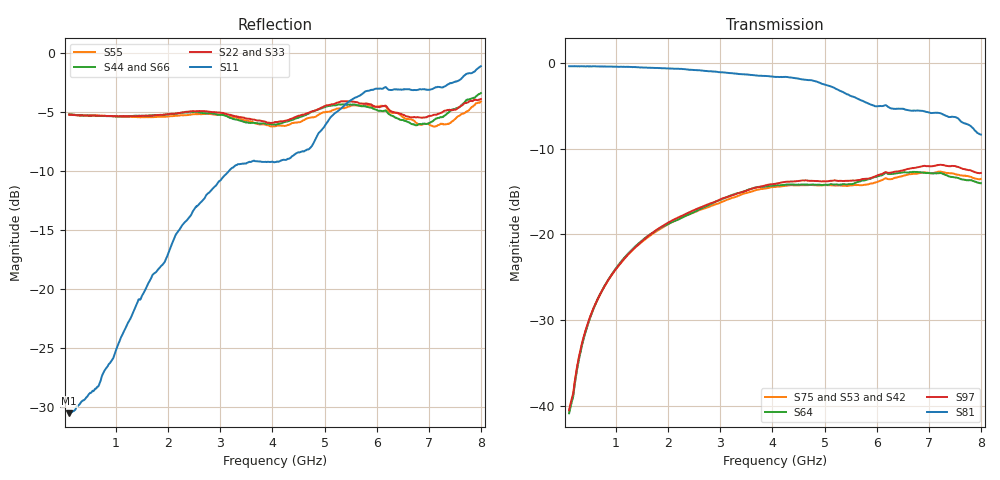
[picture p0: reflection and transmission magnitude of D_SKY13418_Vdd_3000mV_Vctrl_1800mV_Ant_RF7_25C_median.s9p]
# GHz S DB R 50
! THRU S21 mag phase subtraction.
! HALF_THRU
! EN33-165-011-v1_HALF_THRU_1 EN33-165-011-v1_HALF_THRU_2 EN33-165-011-v1_HALF_THRU_3 EN33-165-011-v1_HALF_THRU_4 EN33-165-011-v1_HALF_THRU_5 EN33-165-011-v1_HALF_THRU_6 EN33-165-011-v1_HALF_THRU_7 EN33-165-011-v1_HALF_THRU_8 EN33-165-011-v1_HALF_THRU_9
! THRU Ports: 1 2
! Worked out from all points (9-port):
!   801 points, 100 MHz to 8 GHz, reference 50 ohm
!   strongest paths, dB at 100 MHz, 2.075 GHz, 4.05 GHz, 6.025 GHz, 8 GHz:
!     S81: -0.4, -0.7, -1.6, -5.0, -8.3
!     S97: -40.5, -18.4, -14.1, -13.1, -12.8
!     S64: -40.9, -18.6, -14.3, -13.2, -14.0
!     S75: -40.6, -18.6, -14.4, -13.8, -13.5
!     S53: -41.0, -18.8, -14.6, -13.8, -13.6
!     S42: -41.0, -18.9, -14.7, -13.5, -13.8
!   lowest |S11| = -30.5 dB at 100 MHz (marker M1), VSWR 1.06, Z = 53.1 - j0.109 ohm
!   |S11| at or under -10 dB: start of sweep to 3.162 GHz
